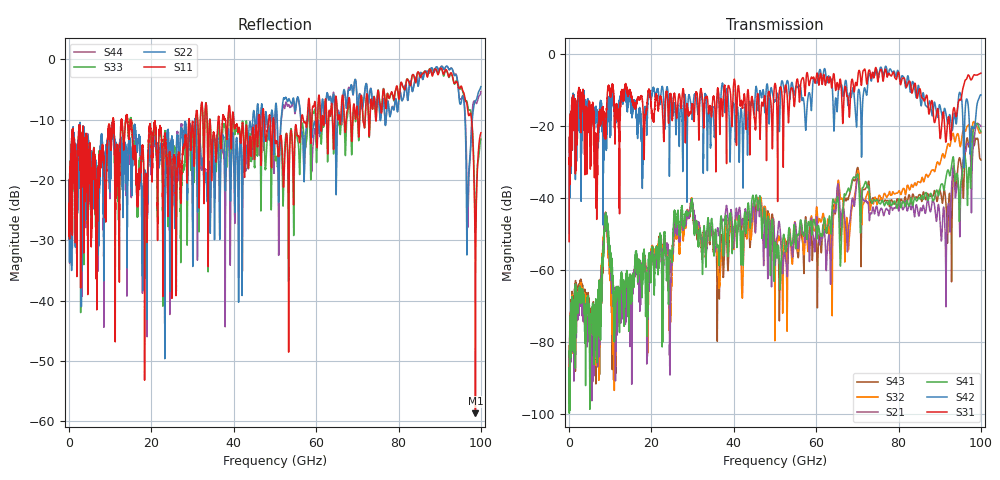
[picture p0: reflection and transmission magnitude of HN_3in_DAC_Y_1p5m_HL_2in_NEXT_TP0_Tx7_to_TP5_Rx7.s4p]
# GHz S RI R 45
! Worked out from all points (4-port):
!   4000 points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, 25 MHz to 100 GHz, reference 45 ohm
!   strongest paths, dB at 25 MHz, 25.02 GHz, 50.02 GHz, 75.03 GHz, 100 GHz:
!     S31: -52.3, -17.7, -8.3, -7.8, -5.4
!     S42: -50.1, -13.8, -13.1, -6.4, -11.5
!     S41: -87.4, -57.8, -52.9, -40.9, -21.7
!     S21: -95.0, -56.6, -58.2, -44.5, -20.2
!     S32: -98.6, -59.9, -67.8, -40.7, -21.9
!     S43: -97.3, -57.2, -53.5, -40.7, -29.6
!   lowest |S11| = -58.7 dB at 98.67 GHz (marker M1), VSWR 1.00, Z = 44.9 - j0.0587 ohm
!   |S11| at or under -10 dB: start of sweep to 10.66 GHz; 14.21 GHz to 29.11 GHz (14.89 GHz wide, 68.8 % of centre); 49.71 GHz to 56.41 GHz (6.696 GHz wide, 12.6 % of centre)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
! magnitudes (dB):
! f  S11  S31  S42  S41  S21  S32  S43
! 25 MHz  -25.3  -52.3  -50.1  -87.4  -95.0  -98.6  -97.3
! 8.975 GHz  -25.5  -19.8  -19.7  -44.6  -44.7  -44.7  -44.8
! 11 GHz  -13.1  -16.2  -15.2  -71.4  -67.9  -93.6  -86.4
! 29.6 GHz  -14.9  -16.3  -14.0  -42.8  -41.1  -40.9  -41.8
! 91.5 GHz  -1.7  -24.6  -16.6  -34.6  -66.5  -27.4  -41.4
! 98.67 GHz  -58.7  -6.0  -18.7  -19.8  -20.9  -19.8  -23.7
! 100 GHz  -12.2  -5.4  -11.5  -21.7  -20.2  -21.9  -29.6
